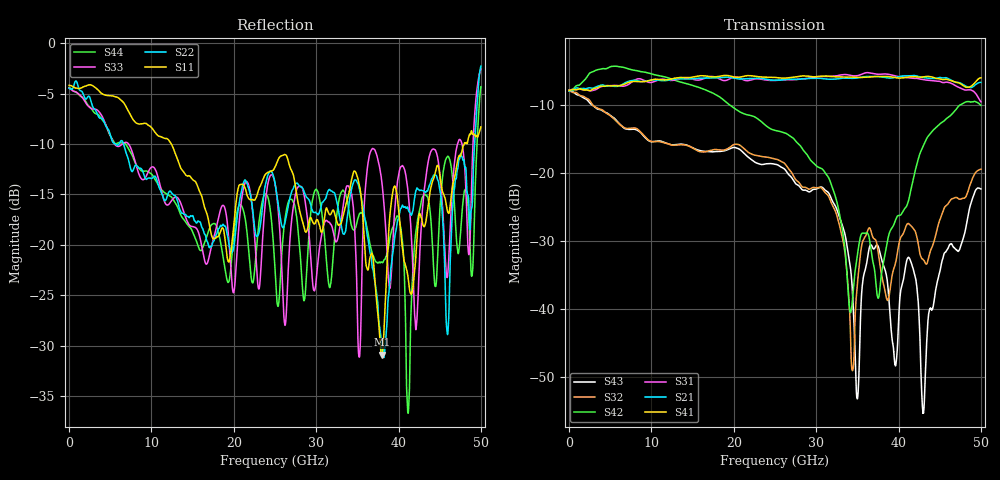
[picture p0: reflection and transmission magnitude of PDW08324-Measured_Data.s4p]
!Keysight Technologies,N5227B,US57180409,A.13.20.10
!Date: Wednesday, July 17, 2019 10:57:09
!Correction: S11(Full 4 Port(1,2,3,4))
!S12(Full 4 Port(1,2,3,4))
!S13(Full 4 Port(1,2,3,4))
!S14(Full 4 Port(1,2,3,4))
!S21(Full 4 Port(1,2,3,4))
!S22(Full 4 Port(1,2,3,4))
!S23(Full 4 Port(1,2,3,4))
!S24(Full 4 Port(1,2,3,4))
!S31(Full 4 Port(1,2,3,4))
!S32(Full 4 Port(1,2,3,4))
!S33(Full 4 Port(1,2,3,4))
!S34(Full 4 Port(1,2,3,4))
!S41(Full 4 Port(1,2,3,4))
!S42(Full 4 Port(1,2,3,4))
!S43(Full 4 Port(1,2,3,4))
!S44(Full 4 Port(1,2,3,4))
!S4P File: Measurements: <S11,S12,S13,S14>,
!<S21,S22,S23,S24>,
!<S31,S32,S33,S34>,
!<S41,S42,S43,S44>:
# Hz S  dB  R 50
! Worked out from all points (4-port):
!   5000 points, 10 MHz to 50 GHz, reference 50 ohm
!   strongest paths, dB at 10 MHz, 12.51 GHz, 25.01 GHz, 37.51 GHz, 50 GHz:
!     S41: -7.9, -6.2, -6.0, -5.9, -6.1
!     S21: -8.0, -6.3, -6.4, -5.9, -6.7
!     S31: -7.9, -6.4, -6.4, -5.5, -9.6
!     S42: -7.9, -6.3, -13.8, -38.4, -10.1
!     S32: -8.0, -16.0, -18.0, -31.6, -19.5
!     S43: -7.9, -15.9, -18.8, -30.8, -22.4
!   lowest |S11| = -30.9 dB at 37.97 GHz (marker M1), VSWR 1.06, Z = 52.9 + j0.522 ohm
!   |S11| at or under -10 dB: 12.42 GHz to 47.97 GHz (35.55 GHz wide, 118 % of centre)
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1e7  -4.19 179.5  -8.00 -0.3  -7.85 -0.7  -7.89 -0.6
     -8.00 -0.2  -4.49 178.6  -8.03 -1.8  -7.86 0.5
     -7.88 -0.5  -8.02 -1.9  -4.44 177.7  -7.94 -2.1
     -7.90 -0.6  -7.87 0.4  -7.95 -2.4  -4.40 178.2
3.138e10  -16.57 -100.0  -6.25 -119.9  -5.87 -134.6  -5.81 -137.6
          -6.26 -119.8  -14.78 -109.5  -23.24 64.6  -20.47 32.7
          -5.87 -134.6  -23.25 64.5  -17.64 -147.2  -22.79 36.9
          -5.81 -137.5  -20.48 32.6  -22.80 36.9  -22.83 -109.6
3.498e10  -13.18 -14.9  -6.08 -179.2  -5.74 159.8  -6.01 160.7
          -6.09 -179.1  -13.81 -150.1  -36.72 97.3  -32.29 140.5
          -5.75 159.8  -36.76 97.7  -25.71 -145.1  -53.46 -20.4
          -6.01 160.8  -32.34 140.2  -53.22 149.6  -17.67 150.5
3.797e10  -30.88 9.9  -5.93 128.1  -5.52 105.6  -5.85 107.6
          -5.94 128.1  -30.39 169.6  -35.27 3.7  -34.53 161.1
          -5.52 105.6  -35.19 3.6  -13.74 133.7  -32.76 -81.0
          -5.85 107.6  -34.57 161.1  -32.82 -81.7  -21.75 100.2
4.299e10  -18.06 69.6  -6.00 36.3  -6.31 9.9  -5.91 15.3
          -6.00 36.3  -14.62 -54.0  -32.80 -49.7  -16.11 157.0
          -6.31 9.9  -32.75 -49.4  -15.69 -47.8  -55.83 -8.3
          -5.91 15.3  -16.12 157.1  -55.31 99.6  -15.13 63.0
4.595e10  -16.68 64.0  -6.13 -25.2  -6.71 -48.2  -6.31 -44.2
          -6.13 -25.2  -28.89 -131.9  -24.65 -83.0  -11.93 106.1
          -6.71 -48.3  -24.66 -83.0  -23.15 -5.4  -31.20 -84.5
          -6.32 -44.1  -11.93 106.2  -31.23 -83.9  -11.23 44.2
5e10  -8.31 -12.5  -6.71 -118.3  -9.59 -141.1  -6.04 -132.9
      -6.73 -118.1  -2.29 -100.8  -19.45 146.8  -10.10 6.4
      -9.58 -141.0  -19.49 146.3  -2.60 -96.8  -22.45 174.5
      -6.06 -133.1  -10.11 6.2  -22.39 174.6  -4.32 -98.8
